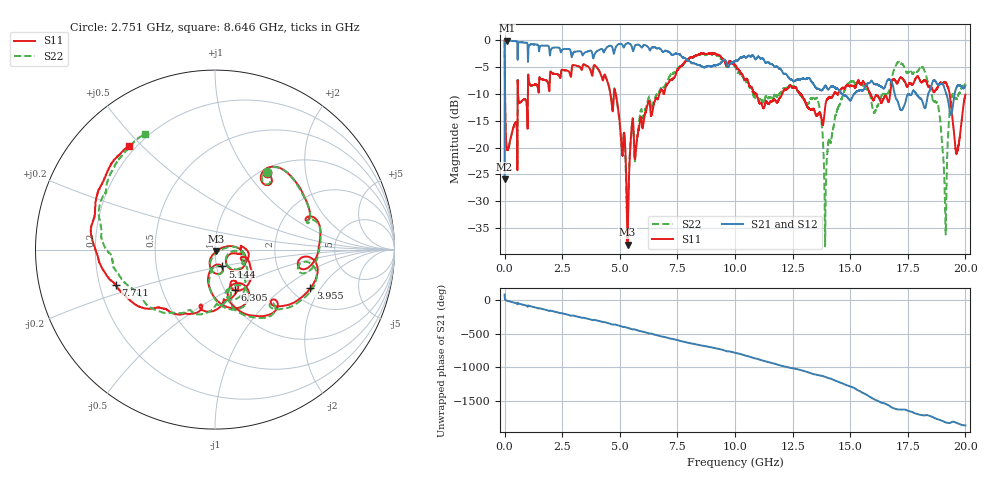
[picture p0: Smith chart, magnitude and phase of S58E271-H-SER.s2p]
!{S58E271}
!Johanson Technology Inc.
!www.johansontechnology.com
!Test Board Conditions:
!Substrate Type  RO4350B
!Substrate Thickness  60 mil
!Substrate Dk  3.66
!TL Type: GCPW
!TL Trace Width  115 mil
!TL Gap  52 mil
!Electrode orientation  Horizontal
!DUT TOPOLOGY	SERIES
!Mounting Pad LxW  55x428 mil
! Created Wed Apr 14 11:38:42 2021
# mhz S ma R 50
! 2 Port Network Data from SP1.SP block
! freq  magS11  angS11  magS21  angS21  magS12  angS12  magS22  angS22
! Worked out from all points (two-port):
!   20001 points, 300 kHz to 20 GHz, reference 50 ohm
!   highest |S21| = -0.05 dB at 107.3 MHz (marker M1); lowest = -25.9 dB at 300 kHz (marker M2)
!   |S21| within 3 dB of the highest: 1.022 GHz to 2.904 GHz (1.882 GHz wide, 95.9 % of centre); 3.875 GHz to 7.688 GHz (3.813 GHz wide, 65.9 % of centre)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
!   lowest |S11| = -38.1 dB at 5.334 GHz (marker M3), VSWR 1.03, Z = 50.8 - j0.997 ohm
!   |S11| at or under -10 dB: 4.826 GHz to 6.719 GHz (1.892 GHz wide, 32.8 % of centre); 10.92 GHz to 12.05 GHz (1.129 GHz wide, 9.83 % of centre); 12.86 GHz to 14.29 GHz (1.435 GHz wide, 10.6 % of centre)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
!   |S22| runs from -38.4 to 0.0 dB; largest |S21 - S12| = 0.013
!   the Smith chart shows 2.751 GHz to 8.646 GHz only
!   S11 on the Smith chart (normalised r, x): 2.751 GHz: 1.07, +1.25; 3.955 GHz: 2.53, -1.62; 5.144 GHz: 1.06, -0.20; 6.305 GHz: 1.11, -0.54; 7.711 GHz: 0.27, -0.16; 8.646 GHz: 0.17, +0.46
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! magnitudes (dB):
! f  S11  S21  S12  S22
! 300 kHz  0.0  -25.9  -25.9  0.0
! 107.3 MHz  -20.4  -0.1  -0.1  -20.4
! 2.751 GHz  -5.7  -1.6  -1.6  -5.7
! 3.334 GHz  -5.4  -2.2  -2.2  -5.4
! 3.955 GHz  -4.8  -2.3  -2.2  -4.8
! 5.144 GHz  -19.8  -1.2  -1.2  -19.0
! 5.334 GHz  -38.1  -0.5  -0.5  -33.7
! 5.522 GHz  -15.8  -1.2  -1.2  -15.7
! 6.305 GHz  -12.0  -1.9  -1.9  -10.8
! 6.667 GHz  -10.8  -1.4  -1.5  -10.2
! 7.711 GHz  -4.6  -3.2  -3.2  -4.8
! 8.646 GHz  -2.5  -5.0  -5.1  -2.5
! 10 GHz  -4.6  -3.8  -3.8  -4.9
! 13.33 GHz  -12.9  -7.8  -7.8  -10.9
! 13.93 GHz  -11.8  -8.5  -8.6  -29.3
! 14.9 GHz  -8.3  -10.7  -10.6  -8.2
! 16.67 GHz  -11.4  -7.3  -7.4  -9.7
! 18.19 GHz  -7.5  -12.2  -12.1  -5.2
! 18.83 GHz  -8.4  -8.3  -8.3  -12.6
! 19.12 GHz  -7.8  -9.3  -9.2  -31.4
! 19.63 GHz  -20.8  -8.6  -8.5  -10.9
! 20 GHz  -10.1  -8.4  -8.4  -8.3
